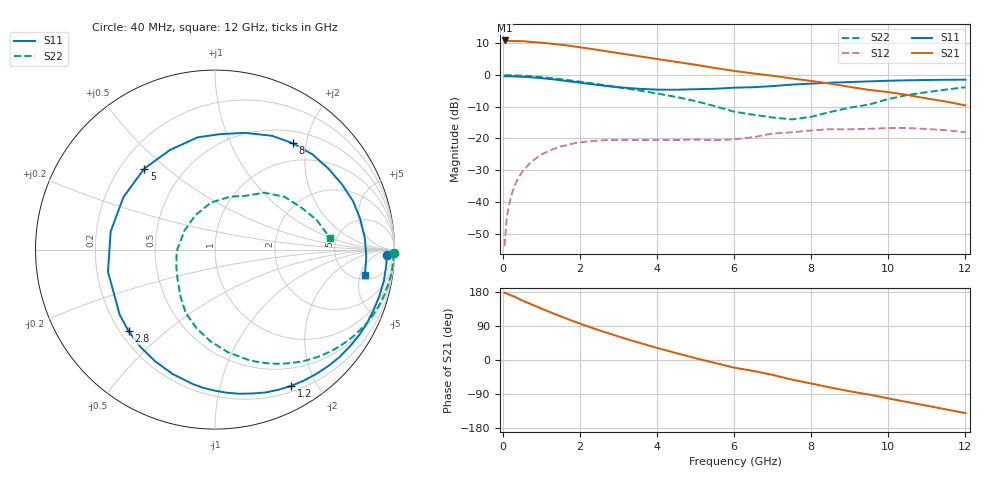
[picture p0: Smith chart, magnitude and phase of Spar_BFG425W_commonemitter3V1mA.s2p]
! Filename: 31bfg425.001
! BFG425W Field C1
! V1=7.859E-001V,V2=3.000E+000V, I1=1.141E-005A, I2=1.000E-003A
# GHz  S  MA  R 50
!  S11  S21  S12  S22
!Freq(GHz)  Mag  Ang  Mag  Ang  Mag  Ang  Mag  Ang
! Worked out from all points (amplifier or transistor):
!   44 points, 40 MHz to 12 GHz, reference 50 ohm
!   highest |S21| = 10.9 dB at 40 MHz (marker M1)
!   |S21| within 3 dB of that: start of sweep to 2.466 GHz
!   unconditionally stable (mu >= 1): 3.398 GHz to end of sweep
!   at 700 MHz: K = 0.12, MSG = 19.1 dB, |S12| = -27.7 dB
!   at 2.4 GHz: K = 0.56, MSG = 14.4 dB, |S12| = -20.7 dB
!   at 12 GHz: K = 2.20, MAG = -2.0 dB, |S12| = -18.1 dB
!   S11 on the Smith chart (normalised r, x): 40 MHz: 29, -23; 1.2 GHz: 0.27, -1.67; 2.8 GHz: 0.23, -0.38; 5 GHz: 0.30, +0.42; 8 GHz: 0.69, +1.76; 12 GHz: 5.98, -5.99
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0.04  0.958 -1.9  3.52 177.6  0.002 71.7  0.996 -1.2
0.1  0.958 -5.2  3.458 175.3  0.006 86.4  0.995 -3.0
0.2  0.957 -10.3  3.451 170.7  0.012 82.1  0.993 -5.9
0.3  0.952 -15.5  3.441 166.9  0.018 78.7  0.99 -8.8
0.5  0.941 -25.7  3.43 157.1  0.03 71.7  0.978 -14.6
0.7  0.925 -35.8  3.344 148.4  0.041 64.7  0.961 -20.2
1  0.893 -50.9  3.243 135.4  0.056 54.6  0.927 -28.4
1.2  0.87 -60.8  3.152 127.1  0.064 48.2  0.902 -33.6
1.7  0.8 -85.3  2.917 107.2  0.08 33.6  0.831 -45.8
2.2  0.732 -108.9  2.634 88.7  0.09 20.9  0.756 -56.9
2.8  0.662 -136.7  2.319 68.3  0.095 8.6  0.67 -69.1
3.5  0.609 -168.3  1.997 46.5  0.095 -2.1  0.576 -82.9
4  0.59 170.1  1.793 31.7  0.095 -7.9  0.512 -92.7
4.5  0.588 150.1  1.614 18.1  0.095 -11.8  0.451 -103.1
5  0.599 131.1  1.452 4.6  0.096 -16.6  0.388 -114.9
6  0.633 98.8  1.163 -20.2  0.097 -23.7  0.264 -142.4
6.5  0.644 87.4  1.061 -28.9  0.105 -17.5  0.237 -155.2
7.5  0.709 63.5  0.884 -51.9  0.125 -32.8  0.2 147.8
8  0.734 53.8  0.808 -62.0  0.134 -38.6  0.22 120.3
8.5  0.759 44.4  0.732 -72.8  0.14 -47.2  0.263 94.8
10.5  0.827 12.0  0.485 -111.1  0.146 -81.3  0.486 37.4
12  0.847 -9.6  0.332 -140.1  0.125 -113.3  0.644 5.7
